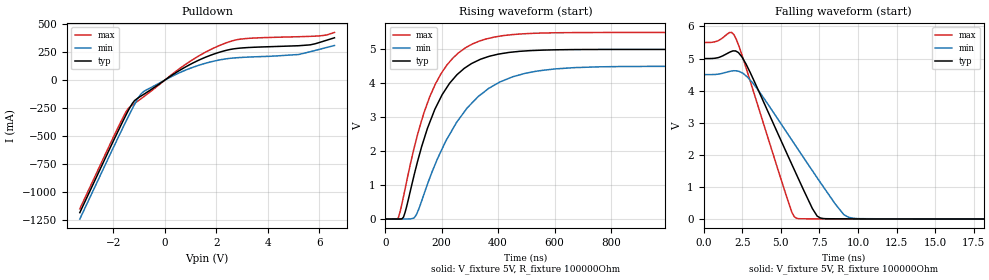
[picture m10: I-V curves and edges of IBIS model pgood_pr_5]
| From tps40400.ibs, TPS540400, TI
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|   pgood_pr_5 Model
[Model]   pgood_pr_5
Model_type   Open_drain
Polarity   Non-Inverting
Vmeas = 2.5
Vref = 5
Cref = 1pF
Rref = 100000
|   typ   min   max
C_comp   1.431pF   1.292pF   1.756pF
[Voltage Range]   3.3   3.2   3.4
[Temperature Range]   25   125   -40
[Pullup Reference]   3.3   3.2   3.4
[Pulldown Reference]   -0   -0   -0
[Power Clamp Reference]   3.3   3.2   3.4
[GND Clamp Reference]   -0   -0   -0
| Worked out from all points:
|   slope of the pulldown table from 0 to 0.495 V, typ, clamps not added: 6.57 ohm
|   falling waveform, V_fixture 5V, R_fixture 100000Ohm: 20-80 % time 2.83ns typ, 3.78ns min, 2.16ns max; typ from 5 V to 0 V
|   rising waveform, V_fixture 5V, R_fixture 100000Ohm: 20-80 % time 134ns typ, 184ns min, 132ns max; typ from 0 V to 5 V
[Pulldown]
|   Voltage   I(typ)   I(min)   I(max)
-3.3V     -1.181A    -1.238A    -1.147A
-1.518V   -316.1mA   -372.4mA   -288mA
-1.379V   -254.8mA   -308mA     -243.1mA
-1.171V   -181.7mA   -215.2mA   -207.3mA
-825mV    -127.7mA   -102mA     -149.2mA
976.8mV   138.9mA    104.5mA    166.5mA
1.769V    221mA      161.9mA    271.1mA
2.501V    271.5mA    193.4mA    341.5mA
3.194V    289.9mA    204.9mA    371.3mA
5.194V    306.5mA    228.3mA    386.9mA
5.848V    324.5mA    264.9mA    392.1mA
6.59V     377.4mA    308.9mA    424.9mA
[Ramp]
R_load = 100000
|   typ   min   max
dV/dt_r   2.9998/1.34179e-07   2.69976/1.8401e-07   3.29981/1.31542e-07
dV/dt_f   2.9998/2.83027e-09   2.69976/3.77631e-09   3.29981/2.1579e-09
[Falling Waveform]
V_fixture = 5V
V_fixture_min = 4.5V
V_fixture_max = 5.5V
R_fixture = 100000Ohm
C_fixture = 0F
|   Time   V(typ)   V(min)   V(max)
0s        5V         4.5V       5.5V
1.821ns   5.224V     4.612V     5.812V
2.473ns   5.058V     4.558V     5.124V
3.565ns   3.992V     3.996V     3.459V
5.718ns   1.702V     2.46V      213.3mV
7.054ns   322.3mV    1.502V     6.773mV
7.644ns   26.24mV    1.085V     4.533mV
9.382ns   5.806mV    56.89mV    3.086mV
14.89ns   2.662mV    3.732mV    1.948mV
3us       335.5uV    395.8uV    314.2uV
[Rising Waveform]
V_fixture = 5V
V_fixture_min = 4.5V
V_fixture_max = 5.5V
R_fixture = 100000Ohm
C_fixture = 0F
|   Time   V(typ)   V(min)   V(max)
0s        335.5uV    395.8uV    314.2uV
42.66ns   366.3uV    91.89uV    2.161mV
64.33ns   56.12mV    1.026mV    662.5mV
109.7ns   1.55V      121.1mV    2.344V
157ns     2.839V     1.198V     3.596V
197.7ns   3.603V     2.004V     4.288V
290.7ns   4.502V     3.279V     5.078V
388.3ns   4.837V     3.956V     5.367V
752.6ns   4.999V     4.486V     5.499V
3us       5V         4.5V       5.5V
